| TEXAS INSTRUMENTS INCORPORATED
| Standard Linear and Logic Group
| IBIS Model of SN74ALVCH162721
| 3.3-V 20-BIT FLIP-FLOP WITH 3-STATE OUTPUTS
| This file contains package information for the following:
|  TSSOP 56-pin (DGG) package as [Component] ALVCH162721_DGG
|  SSOP 56-pin (DL) package as [Component] ALVCH162721_DL
| This device can be powered at the following Vccs:
|  1.8 volt Vcc
|  2.5 volt Vcc
|  3.3 volt Vcc
| This file provides unique models under the [Model Selector] for each Vcc.
| For operation at a specific Vcc, select the appropriate model after each
| [Model Selector] keyword.
[IBIS Ver]   3.2
[Comment char]  |_char
[File Name]   sn74alvch162721.ibs
[File Rev]   1.1 | b_die
[Date]   March 26, 2003
[Source]   Data created from TI-SPICE simulations at TI-SLL.
[Notes]   The following is an IBIS list for the SN74ALVCH162721.
   Please contact sllibis@ti.com with questions and
   comments concerning SLL IBIS models.
   This IBIS model is created from a BA (back annotated
   netlist).
   - C_comp values are taken at a different test condition than
   the Ci and Co in data sheet.
   - Non-monotonic data in ground-clamp due to bus-hold
   - Non-monotonic data in pullup/pulldown data due to
   damping resistor.
[Disclaimer] Property of Texas Instruments Incorporated. Unauthorized
   reproduction and/or distribution is strictly prohibited.
   This product is protected under copyright law.
   Created 2003,(C) Copyright 2003, Texas Instruments
   Incorporated, All Rights Reserved
   UNLESS THERE IS A SIGNED, WRITTEN AGREEMENT TO THE
   CONTRARY, TEXAS INSTRUMENTS (TI) IS PROVIDING THE IBIS
   MODELS AND WITHOUT ANY WARRANTY, EXPRESSED OR
   IMPLIED. TI assumes no liability for:
   1) the accuracy of the IBIS models provided to your
   company;
   2) the proper functioning of these IBIS Models in your
   design or for any resulting applications; or
   3) infringement of patents, copyrights or intellectual
   property rights resulting from your use of these IBIS
   models.
   TI provides IBIS Models as a service to our customers.
   You and your company shall not distribute, sell or give
   these models to anyone else without prior written
   permission from TI.
   TI reserves the right to make changes to our products or
   to discontinue any semiconductor product or service
   without notice, and advises our customers to obtain the
   latest version of relevant information to verify, before
   placing orders, that the information being relied on is
   current.
   Please be aware that your receipt and use of the IBIS
   information provided shall serve as acceptance of these
   terms and conditions. If you do not accept these terms,
   you should return or destroy the IBIS models and any
   other accompanying information immediately.
| Component ALVCH162721_DGG 56-pin TSSOP
[Component]   ALVCH162721_DGG
[Manufacturer]   Texas Instruments, Inc.
[Package]
|   typ   min   max
R_pkg   4.500e-02   3.500e-02   6.200e-02
L_pkg   3.324e-09   2.403e-09   5.094e-09
C_pkg   5.640e-13   3.410e-13   9.140e-13
[Pin]   signal_name   model_name   R_pin   L_pin   C_pin
1   NOE   ALVCH162721_OE   6.200e-02   5.094e-09   8.560e-13
2   Q1   ALVCH162721_OUT   6.100e-02   4.621e-09   9.020e-13
3   Q2   ALVCH162721_OUT   6.000e-02   4.316e-09   8.020e-13
4   GND   GND   5.900e-02   3.968e-09   6.980e-13
5   Q3   ALVCH162721_OUT   5.700e-02   3.716e-09   6.490e-13
6   Q4   ALVCH162721_OUT   4.200e-02   3.517e-09   6.530e-13
7   VCC   POWER   4.100e-02   3.160e-09   5.700e-13
8   Q5   ALVCH162721_OUT   3.900e-02   2.981e-09   4.820e-13
9   Q6   ALVCH162721_OUT   3.900e-02   2.808e-09   4.470e-13
10   Q7   ALVCH162721_OUT   3.800e-02   2.715e-09   4.090e-13
11   GND   GND   4.100e-02   2.675e-09   3.910e-13
12   Q8   ALVCH162721_OUT   3.900e-02   2.536e-09   3.660e-13
13   Q9   ALVCH162721_OUT   3.900e-02   2.457e-09   3.480e-13
14   Q10   ALVCH162721_OUT   3.800e-02   2.411e-09   3.530e-13
15   Q11   ALVCH162721_OUT   3.900e-02   2.456e-09   3.550e-13
16   Q12   ALVCH162721_OUT   3.900e-02   2.471e-09   3.490e-13
17   Q13   ALVCH162721_OUT   4.000e-02   2.580e-09   3.700e-13
18   GND   GND   3.800e-02   2.651e-09   3.890e-13
19   Q14   ALVCH162721_OUT   3.800e-02   2.739e-09   4.110e-13
20   Q15   ALVCH162721_OUT   3.900e-02   2.838e-09   4.490e-13
21   Q16   ALVCH162721_OUT   3.800e-02   2.988e-09   4.840e-13
22   VCC   POWER   3.800e-02   3.104e-09   5.640e-13
23   Q17   ALVCH162721_OUT   4.000e-02   3.427e-09   6.380e-13
24   Q18   ALVCH162721_OUT   5.600e-02   3.654e-09   6.410e-13
25   GND   GND   5.700e-02   3.932e-09   7.000e-13
26   Q19   ALVCH162721_OUT   5.800e-02   4.257e-09   8.060e-13
27   Q20   ALVCH162721_OUT   5.700e-02   4.580e-09   9.140e-13
28   NC   NC   5.900e-02   5.038e-09   8.610e-13
29   NCLKEN   ALVCH162721_CE   6.000e-02   5.058e-09   8.580e-13
30   D20   ALVCH162721_IN   5.600e-02   4.543e-09   9.040e-13
31   D19   ALVCH162721_IN   5.700e-02   4.241e-09   8.020e-13
32   GND   GND   5.900e-02   3.933e-09   6.990e-13
33   D18   ALVCH162721_IN   5.600e-02   3.616e-09   6.370e-13
34   D17   ALVCH162721_IN   3.700e-02   3.368e-09   6.400e-13
35   VCC   POWER   3.600e-02   3.024e-09   5.630e-13
36   D16   ALVCH162721_IN   3.500e-02   2.876e-09   4.740e-13
37   D15   ALVCH162721_IN   3.500e-02   2.745e-09   4.440e-13
38   D14   ALVCH162721_IN   3.700e-02   2.683e-09   4.050e-13
39   GND   GND   3.800e-02   2.603e-09   3.820e-13
40   D13   ALVCH162721_IN   3.800e-02   2.510e-09   3.620e-13
41   D12   ALVCH162721_IN   3.600e-02   2.412e-09   3.410e-13
42   D11   ALVCH162721_IN   3.800e-02   2.416e-09   3.490e-13
43   D10   ALVCH162721_IN   3.800e-02   2.403e-09   3.490e-13
44   D9   ALVCH162721_IN   3.700e-02   2.429e-09   3.410e-13
45   D8   ALVCH162721_IN   3.600e-02   2.483e-09   3.580e-13
46   GND   GND   3.700e-02   2.614e-09   3.810e-13
47   D7   ALVCH162721_IN   3.500e-02   2.669e-09   4.020e-13
48   D6   ALVCH162721_IN   3.600e-02   2.763e-09   4.420e-13
49   D5   ALVCH162721_IN   3.600e-02   2.942e-09   4.780e-13
50   VCC   POWER   3.500e-02   3.053e-09   5.640e-13
51   D4   ALVCH162721_IN   3.600e-02   3.408e-09   6.410e-13
52   D3   ALVCH162721_IN   5.800e-02   3.698e-09   6.410e-13
53   GND   GND   5.900e-02   3.974e-09   6.970e-13
54   D2   ALVCH162721_IN   6.100e-02   4.327e-09   8.020e-13
55   D1   ALVCH162721_IN   6.100e-02   4.624e-09   9.050e-13
56   CLK   ALVCH162721_CLK   6.000e-02   5.063e-09   8.580e-13
| Component ALVCH162721_DL 56-pin SSOP
[Component]   ALVCH162721_DL
[Manufacturer]   Texas Instruments, Inc.
[Package]
|   typ   min   max
R_pkg   5.500e-02   4.800e-02   6.700e-02
L_pkg   6.539e-09   4.803e-09   9.746e-09
C_pkg   8.570e-13   5.000e-13   1.351e-12
[Pin]   signal_name   model_name   R_pin   L_pin   C_pin
1   NOE   ALVCH162721_OE   6.400e-02   9.646e-09   1.202e-12
2   Q1   ALVCH162721_OUT   5.900e-02   8.723e-09   1.348e-12
3   Q2   ALVCH162721_OUT   5.900e-02   8.139e-09   1.223e-12
4   GND   GND   5.600e-02   7.554e-09   1.088e-12
5   Q3   ALVCH162721_OUT   5.400e-02   6.991e-09   9.660e-13
6   Q4   ALVCH162721_OUT   5.300e-02   6.659e-09   9.730e-13
7   VCC   POWER   5.500e-02   6.321e-09   9.050e-13
8   Q5   ALVCH162721_OUT   5.600e-02   5.942e-09   7.130e-13
9   Q6   ALVCH162721_OUT   5.700e-02   5.768e-09   6.780e-13
10   Q7   ALVCH162721_OUT   5.400e-02   5.459e-09   6.310e-13
11   GND   GND   5.100e-02   5.224e-09   6.380e-13
12   Q8   ALVCH162721_OUT   4.800e-02   5.088e-09   6.010e-13
13   Q9   ALVCH162721_OUT   5.000e-02   5.021e-09   5.180e-13
14   Q10   ALVCH162721_OUT   5.100e-02   4.803e-09   5.000e-13
15   Q11   ALVCH162721_OUT   5.100e-02   4.803e-09   5.000e-13
16   Q12   ALVCH162721_OUT   5.000e-02   5.021e-09   5.180e-13
17   Q13   ALVCH162721_OUT   4.800e-02   5.088e-09   6.010e-13
18   GND   GND   5.100e-02   5.224e-09   6.380e-13
19   Q14   ALVCH162721_OUT   5.400e-02   5.459e-09   6.310e-13
20   Q15   ALVCH162721_OUT   5.700e-02   5.768e-09   6.770e-13
21   Q16   ALVCH162721_OUT   5.500e-02   5.942e-09   7.150e-13
22   VCC   POWER   5.500e-02   6.321e-09   9.070e-13
23   Q17   ALVCH162721_OUT   5.300e-02   6.659e-09   9.720e-13
24   Q18   ALVCH162721_OUT   5.400e-02   6.991e-09   9.660e-13
25   GND   GND   5.600e-02   7.554e-09   1.087e-12
26   Q19   ALVCH162721_OUT   5.900e-02   8.139e-09   1.223e-12
27   Q20   ALVCH162721_OUT   5.900e-02   8.727e-09   1.351e-12
28   NC   NC   6.700e-02   9.746e-09   1.210e-12
29   NCLKEN   ALVCH162721_CE   6.300e-02   9.630e-09   1.203e-12
30   D20   ALVCH162721_IN   6.000e-02   8.751e-09   1.349e-12
31   D19   ALVCH162721_IN   6.000e-02   8.184e-09   1.224e-12
32   GND   GND   5.600e-02   7.543e-09   1.087e-12
33   D18   ALVCH162721_IN   5.400e-02   7.005e-09   9.690e-13
34   D17   ALVCH162721_IN   5.600e-02   6.714e-09   9.750e-13
35   VCC   POWER   5.800e-02   6.384e-09   9.090e-13
36   D16   ALVCH162721_IN   5.700e-02   5.976e-09   7.170e-13
37   D15   ALVCH162721_IN   5.700e-02   5.743e-09   6.770e-13
38   D14   ALVCH162721_IN   5.400e-02   5.468e-09   6.310e-13
39   GND   GND   5.500e-02   5.329e-09   6.440e-13
40   D13   ALVCH162721_IN   5.200e-02   5.189e-09   6.060e-13
41   D12   ALVCH162721_IN   5.200e-02   5.053e-09   5.190e-13
42   D11   ALVCH162721_IN   5.200e-02   4.825e-09   5.020e-13
43   D10   ALVCH162721_IN   5.400e-02   4.897e-09   5.060e-13
44   D9   ALVCH162721_IN   5.200e-02   5.093e-09   5.210e-13
45   D8   ALVCH162721_IN   5.100e-02   5.179e-09   6.080e-13
46   GND   GND   5.400e-02   5.314e-09   6.450e-13
47   D7   ALVCH162721_IN   5.500e-02   5.511e-09   6.320e-13
48   D6   ALVCH162721_IN   5.700e-02   5.770e-09   6.770e-13
49   D5   ALVCH162721_IN   5.600e-02   5.956e-09   7.160e-13
50   VCC   POWER   5.500e-02   6.320e-09   9.050e-13
51   D4   ALVCH162721_IN   5.200e-02   6.621e-09   9.680e-13
52   D3   ALVCH162721_IN   5.300e-02   6.974e-09   9.660e-13
53   GND   GND   5.700e-02   7.571e-09   1.089e-12
54   D2   ALVCH162721_IN   5.700e-02   8.097e-09   1.219e-12
55   D1   ALVCH162721_IN   5.900e-02   8.723e-09   1.349e-12
56   CLK   ALVCH162721_CLK   6.100e-02   9.560e-09   1.199e-12
| Model ALVCH162721_CLK
[Model Selector]   ALVCH162721_CLK
ALVCH162721_CLK_18   1.8 volt Vcc
ALVCH162721_CLK_25   2.5 volt Vcc
ALVCH162721_CLK_33   3.3 volt Vcc
| Model ALVCH162721_IN
[Model Selector]   ALVCH162721_IN
ALVCH162721_IN_18   1.8 volt Vcc
ALVCH162721_IN_25   2.5 volt Vcc
ALVCH162721_IN_33   3.3 volt Vcc
| Model ALVCH162721_CE
[Model Selector]   ALVCH162721_CE
ALVCH162721_CE_18   1.8 volt Vcc
ALVCH162721_CE_25   2.5 volt Vcc
ALVCH162721_CE_33   3.3 volt Vcc
| Model ALVCH162721_OE
[Model Selector]   ALVCH162721_OE
ALVCH162721_OE_18   1.8 volt Vcc
ALVCH162721_OE_25   2.5 volt Vcc
ALVCH162721_OE_33   3.3 volt Vcc
| Model ALVCH162721_OUT
[Model Selector]   ALVCH162721_OUT
ALVCH162721_OUT_18   1.8 volt Vcc
ALVCH162721_OUT_25   2.5 volt Vcc
ALVCH162721_OUT_33   3.3 volt Vcc
| Models and submodels in the file (15): ALVCH162721_CLK_18 (Input), ALVCH162721_CLK_25 (Input), ALVCH162721_CLK_33 (Input), ALVCH162721_IN_18 (Input), ALVCH162721_IN_25 (Input), ALVCH162721_IN_33 (Input), ALVCH162721_CE_18 (Input), ALVCH162721_CE_25 (Input), ALVCH162721_CE_33 (Input), ALVCH162721_OE_18 (Input), ALVCH162721_OE_25 (Input), ALVCH162721_OE_33 (Input), ALVCH162721_OUT_18 (3-state), ALVCH162721_OUT_25 (3-state), ALVCH162721_OUT_33 (3-state)
